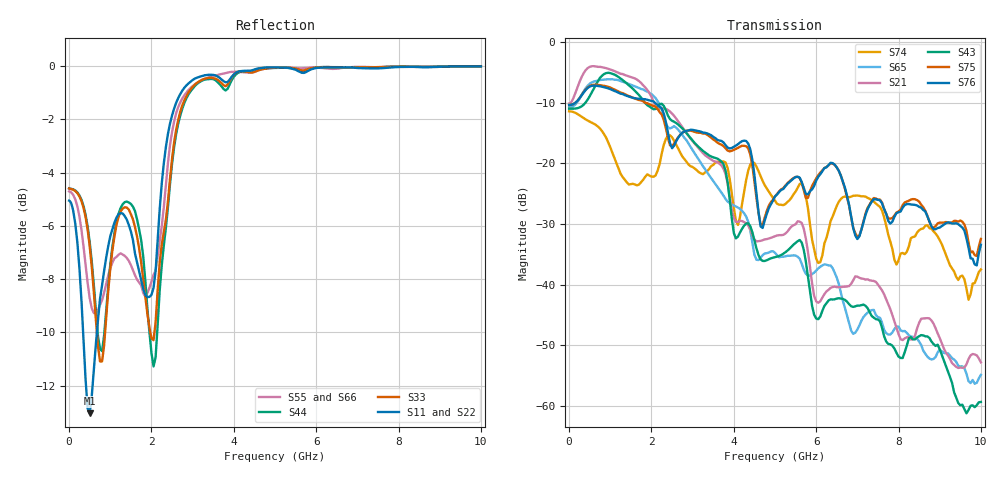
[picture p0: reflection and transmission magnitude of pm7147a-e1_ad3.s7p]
# GHz S DB R 50
! S-Parameters data
! Freq  dbS11  angS11  dbS12  angS12  dbS13  angS13  dbS14  angS14
!  dbS15  angS15  dbS16  angS16  dbS17  angS17  dbS21  angS21
!  dbS22  angS22  dbS23  angS23  dbS24  angS24  dbS25  angS25
!  dbS26  angS26  dbS27  angS27  dbS31  angS31  dbS32  angS32
!  dbS33  angS33  dbS34  angS34  dbS35  angS35  dbS36  angS36
!  dbS37  angS37  dbS41  angS41  dbS42  angS42  dbS43  angS43
!  dbS44  angS44  dbS45  angS45  dbS46  angS46  dbS47  angS47
!  dbS51  angS51  dbS52  angS52  dbS53  angS53  dbS54  angS54
!  dbS55  angS55  dbS56  angS56  dbS57  angS57  dbS61  angS61
!  dbS62  angS62  dbS63  angS63  dbS64  angS64  dbS65  angS65
!  dbS66  angS66  dbS67  angS67  dbS71  angS71  dbS72  angS72
!  dbS73  angS73  dbS74  angS74  dbS75  angS75  dbS76  angS76
!  dbS77  angS77
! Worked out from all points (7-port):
!   279 points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, 1 Hz to 10 GHz, reference 50 ohm
!   strongest paths, dB at 1 Hz, 7.943 MHz, 3.05 GHz, 6.55 GHz, 10 GHz:
!     S76: -10.3, -10.3, -14.5, -21.2, -33.4
!     S75: -10.3, -10.3, -14.8, -21.2, -32.5
!     S43: -11.0, -11.0, -16.6, -42.3, -59.4
!     S21: -10.1, -10.1, -16.7, -40.4, -52.8
!     S65: -10.8, -10.8, -18.3, -39.9, -54.9
!     S74: -11.4, -11.4, -20.8, -26.3, -37.5
!   lowest |S11| = -13.0 dB at 500 MHz (marker M1), VSWR 1.57, Z = 31.8 - j0.651 ohm
!   |S11| at or under -10 dB: 340.9 MHz to 674.6 MHz (333.7 MHz wide, 65.7 % of centre)
